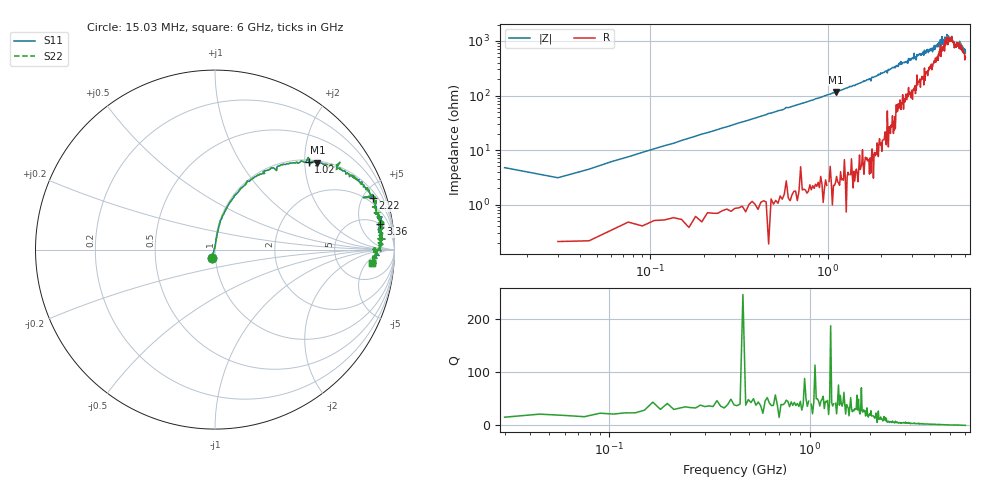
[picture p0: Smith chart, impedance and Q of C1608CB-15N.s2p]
!	Network	Analyzer	HP8753E.07.74:	Oct	30	2002	Serial	No.	JP38451487
!	Hewlett-Packard
!	7	Sep	2009	9:36:41
!	Frequency	S11	S21	S12	S22
#	HZ	S	RI	R	50
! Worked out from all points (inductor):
!   400 points, 15.03 MHz to 6 GHz, reference 50 ohm
!   read as one part in series: L = 15.9 nH near 45.03 MHz
!   highest Q = 48.5 at 1.11 GHz (marker M1), where L = 16.6 nH
!   self-resonance near 5.016 GHz
!   S11 on the Smith chart (normalised r, x): 15.03 MHz: 0.97, -0.09; 1.02 GHz: 1.05, +2.10; 2.22 GHz: 1.52, +5.92; 3.36 GHz: 5, +11; 6 GHz: 11, -7
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1.502992e7  -0.0157 -0.045  1.02 0.045  1.02 0.045  -0.0157 -0.045
3.002985e7  0.00309 0.0308  0.997 -0.0308  0.997 -0.0308  0.00309 0.0308
1.200294e8  0.0193 0.117  0.981 -0.117  0.981 -0.117  0.0193 0.117
3.150284e8  0.0959 0.281  0.904 -0.281  0.904 -0.281  0.0959 0.281
1.020025e9  0.523 0.487  0.477 -0.487  0.477 -0.487  0.523 0.487
1.110024e9  0.571 0.484  0.429 -0.484  0.429 -0.484  0.571 0.484
2.01002e9  0.85 0.331  0.15 -0.331  0.15 -0.331  0.85 0.331
2.220019e9  0.878 0.286  0.122 -0.286  0.122 -0.286  0.878 0.286
3.015015e9  0.93 0.182  0.0705 -0.182  0.0705 -0.182  0.93 0.182
3.360013e9  0.922 0.142  0.0779 -0.142  0.0779 -0.142  0.922 0.142
4.00501e9  0.932 0.09  0.0685 -0.09  0.0685 -0.09  0.932 0.09
4.335008e9  0.927 0.0478  0.0733 -0.0478  0.0733 -0.0478  0.927 0.0478
4.365008e9  0.918 0.0806  0.0817 -0.0806  0.0817 -0.0806  0.918 0.0806
4.425008e9  0.947 0.0584  0.0528 -0.0584  0.0528 -0.0584  0.947 0.0584
4.575007e9  0.908 0.0614  0.0917 -0.0614  0.0917 -0.0614  0.908 0.0614
4.605007e9  0.929 0.0334  0.0707 -0.0334  0.0707 -0.0334  0.929 0.0334
4.665007e9  0.913 0.0359  0.0867 -0.0359  0.0867 -0.0359  0.913 0.0359
4.725006e9  0.935 0.0283  0.0652 -0.0283  0.0652 -0.0283  0.935 0.0283
4.785006e9  0.91 0.0366  0.0896 -0.0366  0.0896 -0.0366  0.91 0.0366
4.815006e9  0.93 0.027  0.0701 -0.027  0.0701 -0.027  0.93 0.027
5.010005e9  0.916 0.0061  0.0843 -0.0061  0.0843 -0.0061  0.916 0.0061
6e9  0.877 -0.0733  0.123 0.0733  0.123 0.0733  0.877 -0.0733
